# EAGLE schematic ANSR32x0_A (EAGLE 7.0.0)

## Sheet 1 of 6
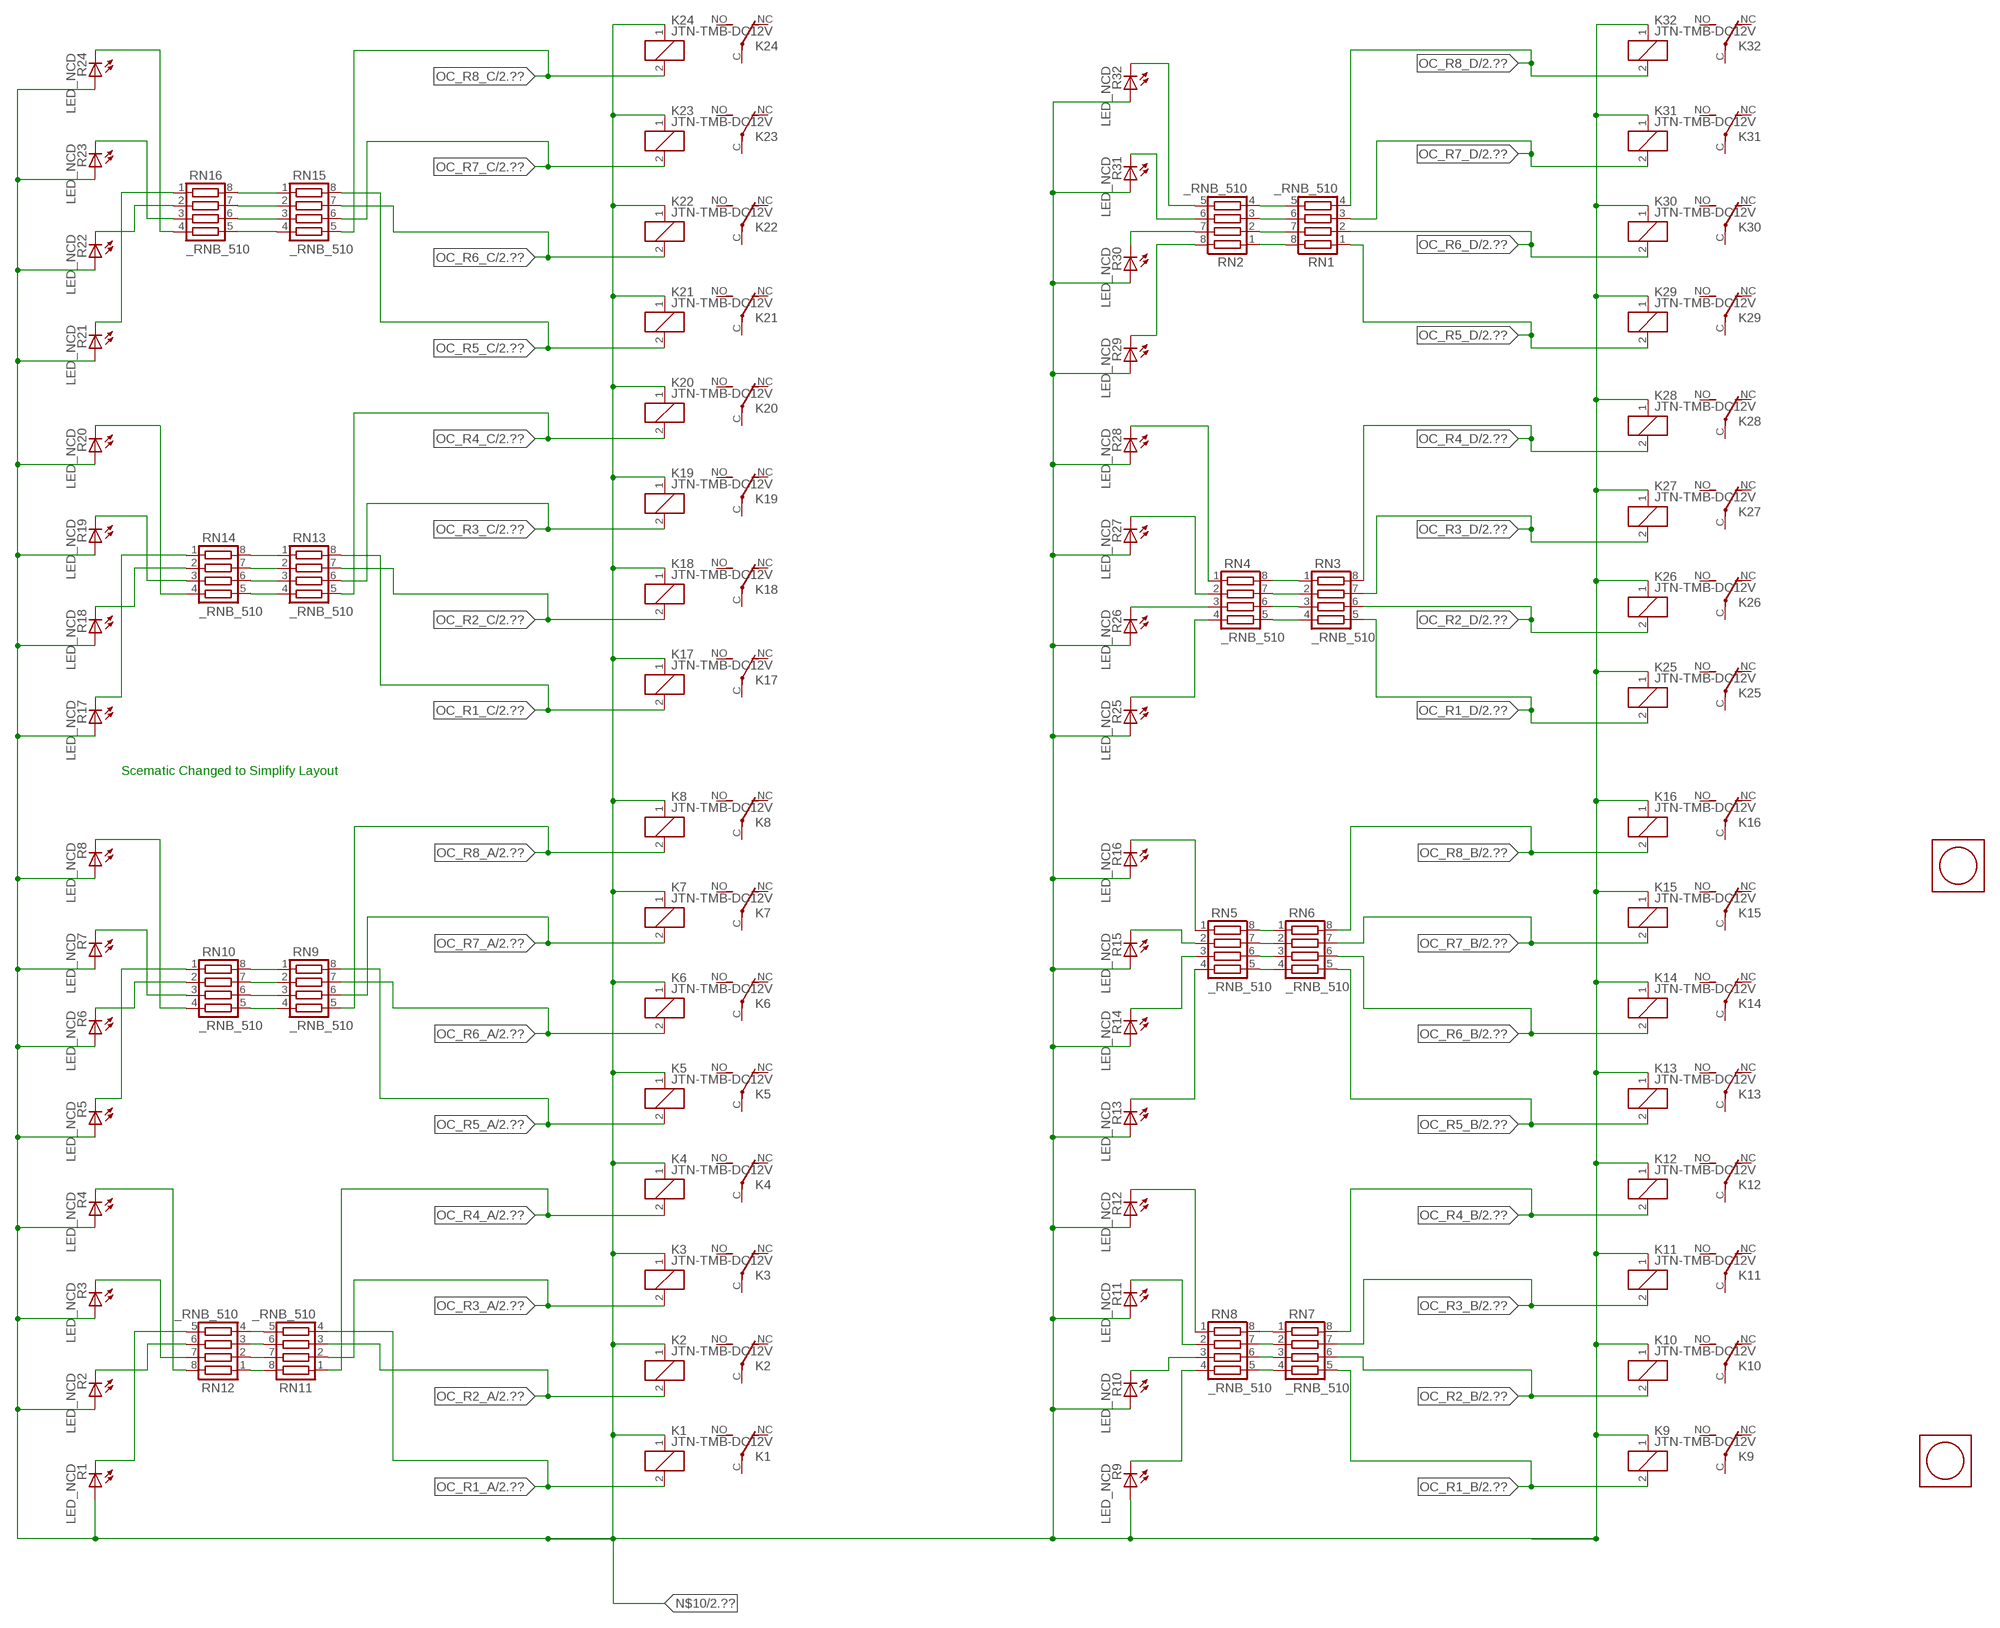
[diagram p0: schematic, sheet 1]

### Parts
K1  JTN-TMB-DC12V  [JT-TMB]
K2  JTN-TMB-DC12V  [JT-TMB]
K3  JTN-TMB-DC12V  [JT-TMB]
K4  JTN-TMB-DC12V  [JT-TMB]
K5  JTN-TMB-DC12V  [JT-TMB]
K6  JTN-TMB-DC12V  [JT-TMB]
K7  JTN-TMB-DC12V  [JT-TMB]
K8  JTN-TMB-DC12V  [JT-TMB]
K9  JTN-TMB-DC12V  [JT-TMB]
K10  JTN-TMB-DC12V  [JT-TMB]
K11  JTN-TMB-DC12V  [JT-TMB]
K12  JTN-TMB-DC12V  [JT-TMB]
K13  JTN-TMB-DC12V  [JT-TMB]
K14  JTN-TMB-DC12V  [JT-TMB]
K15  JTN-TMB-DC12V  [JT-TMB]
K16  JTN-TMB-DC12V  [JT-TMB]
K17  JTN-TMB-DC12V  [JT-TMB]
K18  JTN-TMB-DC12V  [JT-TMB]
K19  JTN-TMB-DC12V  [JT-TMB]
K20  JTN-TMB-DC12V  [JT-TMB]
K21  JTN-TMB-DC12V  [JT-TMB]
K22  JTN-TMB-DC12V  [JT-TMB]
K23  JTN-TMB-DC12V  [JT-TMB]
K24  JTN-TMB-DC12V  [JT-TMB]
K25  JTN-TMB-DC12V  [JT-TMB]
K26  JTN-TMB-DC12V  [JT-TMB]
K27  JTN-TMB-DC12V  [JT-TMB]
K28  JTN-TMB-DC12V  [JT-TMB]
K29  JTN-TMB-DC12V  [JT-TMB]
K30  JTN-TMB-DC12V  [JT-TMB]
K31  JTN-TMB-DC12V  [JT-TMB]
K32  JTN-TMB-DC12V  [JT-TMB]
R1  LED_NCD  [CHIPLED_0603]
R2  LED_NCD  [CHIPLED_0603]
R3  LED_NCD  [CHIPLED_0603]
R4  LED_NCD  [CHIPLED_0603]
R5  LED_NCD  [CHIPLED_0603]
R6  LED_NCD  [CHIPLED_0603]
R7  LED_NCD  [CHIPLED_0603]
R8  LED_NCD  [CHIPLED_0603]
R9  LED_NCD  [CHIPLED_0603]
R10  LED_NCD  [CHIPLED_0603]
R11  LED_NCD  [CHIPLED_0603]
R12  LED_NCD  [CHIPLED_0603]
R13  LED_NCD  [CHIPLED_0603]
R14  LED_NCD  [CHIPLED_0603]
R15  LED_NCD  [CHIPLED_0603]
R16  LED_NCD  [CHIPLED_0603]
R17  LED_NCD  [CHIPLED_0603]
R18  LED_NCD  [CHIPLED_0603]
R19  LED_NCD  [CHIPLED_0603]
R20  LED_NCD  [CHIPLED_0603]
R21  LED_NCD  [CHIPLED_0603]
R22  LED_NCD  [CHIPLED_0603]
R23  LED_NCD  [CHIPLED_0603]
R24  LED_NCD  [CHIPLED_0603]
R25  LED_NCD  [CHIPLED_0603]
R26  LED_NCD  [CHIPLED_0603]
R27  LED_NCD  [CHIPLED_0603]
R28  LED_NCD  [CHIPLED_0603]
R29  LED_NCD  [CHIPLED_0603]
R30  LED_NCD  [CHIPLED_0603]
R31  LED_NCD  [CHIPLED_0603]
R32  LED_NCD  [CHIPLED_0603]
RN1  _RNB_510  [RNB]
RN2  _RNB_510  [RNB]
RN3  _RNB_510  [RNB]
RN4  _RNB_510  [RNB]
RN5  _RNB_510  [RNB]
RN6  _RNB_510  [RNB]
RN7  _RNB_510  [RNB]
RN8  _RNB_510  [RNB]
RN9  _RNB_510  [RNB]
RN10  _RNB_510  [RNB]
RN11  _RNB_510  [RNB]
RN12  _RNB_510  [RNB]
RN13  _RNB_510  [RNB]
RN14  _RNB_510  [RNB]
RN15  _RNB_510  [RNB]
RN16  _RNB_510  [RNB]
U$1  PCB_MOUNTING_HOLE  [PCB_MOUNTING_HOLE]
U$3  PCB_MOUNTING_HOLE  [PCB_MOUNTING_HOLE]

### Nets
N$10: K1.1(C1) K2.1(C1) K3.1(C1) K4.1(C1) K5.1(C1) K6.1(C1) K7.1(C1) K8.1(C1) K9.1(C1) K10.1(C1) K11.1(C1) K12.1(C1) K13.1(C1) K14.1(C1) K15.1(C1) K16.1(C1) K17.1(C1) K18.1(C1) K19.1(C1) K20.1(C1) K21.1(C1) K22.1(C1) K23.1(C1) K24.1(C1) K25.1(C1) K26.1(C1) K27.1(C1) K28.1(C1) K29.1(C1) K30.1(C1) K31.1(C1) K32.1(C1) R1.A R2.A R3.A R4.A R5.A R6.A R7.A R8.A R9.A R10.A R11.A R12.A R13.A R14.A R15.A R16.A R17.A R18.A R19.A R20.A R21.A R22.A R23.A R24.A R25.A R26.A R27.A R28.A R29.A R30.A R31.A R32.A ; also sheet 2
N$440: R30.C RN2.7
N$441: R16.C RN5.1
N$442: RN7.2 RN8.7
N$443: RN7.3 RN8.6
N$444: RN7.4 RN8.5
N$445: R15.C RN5.2
N$446: R26.C RN4.3
N$447: R13.C RN5.4
N$448: RN5.5 RN6.4
N$449: RN7.1 RN8.8
N$450: R12.C RN8.1
N$451: RN5.6 RN6.3
N$452: R11.C RN8.2
N$453: RN5.7 RN6.2
N$454: RN5.8 RN6.1
N$455: RN3.4 RN4.5
N$456: R32.C RN2.5
N$458: R14.C RN5.3
N$459: R10.C RN8.3
N$460: R29.C RN2.8
N$461: R28.C RN4.1
N$462: R27.C RN4.2
N$463: RN11.5 RN12.4
N$464: R25.C RN4.4
N$465: RN1.8 RN2.1
N$466: RN1.7 RN2.2
N$467: RN1.6 RN2.3
N$468: RN1.5 RN2.4
N$469: R31.C RN2.6
N$470: R9.C RN8.4
N$473: R1.C RN12.5
N$474: RN11.6 RN12.3
N$475: R2.C RN12.6
N$476: R3.C RN12.7
N$477: RN9.4 RN10.5
N$478: RN9.3 RN10.6
N$479: RN9.2 RN10.7
N$480: RN9.1 RN10.8
N$481: RN11.7 RN12.2
N$482: R5.C RN10.1
N$483: R4.C RN12.8
N$484: R7.C RN10.3
N$485: R8.C RN10.4
N$486: R6.C RN10.2
N$487: R19.C RN14.3
N$488: R18.C RN14.2
N$489: R17.C RN14.1
N$490: R24.C RN16.4
N$491: RN15.3 RN16.6
N$492: RN15.2 RN16.7
N$493: RN15.1 RN16.8
N$494: R20.C RN14.4
N$495: R23.C RN16.3
N$496: R22.C RN16.2
N$497: R21.C RN16.1
N$500: RN11.8 RN12.1
N$501: RN13.4 RN14.5
N$502: RN13.3 RN14.6
N$503: RN13.2 RN14.7
N$504: RN13.1 RN14.8
N$505: RN3.3 RN4.6
N$506: RN3.2 RN4.7
N$507: RN3.1 RN4.8
N$514: RN15.4 RN16.5
OC_R1_A: K1.2(C2) RN11.4 ; also sheet 2
OC_R1_B: K9.2(C2) RN7.5 ; also sheet 2
OC_R1_C: K17.2(C2) RN13.8 ; also sheet 2
OC_R1_D: K25.2(C2) RN3.5 ; also sheet 2
OC_R2_A: K2.2(C2) RN11.3 ; also sheet 2
OC_R2_B: K10.2(C2) RN7.6 ; also sheet 2
OC_R2_C: K18.2(C2) RN13.7 ; also sheet 2
OC_R2_D: K26.2(C2) RN3.6 ; also sheet 2
OC_R3_A: K3.2(C2) RN11.2 ; also sheet 2
OC_R3_B: K11.2(C2) RN7.7 ; also sheet 2
OC_R3_C: K19.2(C2) RN13.6 ; also sheet 2
OC_R3_D: K27.2(C2) RN3.7 ; also sheet 2
OC_R4_A: K4.2(C2) RN11.1 ; also sheet 2
OC_R4_B: K12.2(C2) RN7.8 ; also sheet 2
OC_R4_C: K20.2(C2) RN13.5 ; also sheet 2
OC_R4_D: K28.2(C2) RN3.8 ; also sheet 2
OC_R5_A: K5.2(C2) RN9.8 ; also sheet 2
OC_R5_B: K13.2(C2) RN6.5 ; also sheet 2
OC_R5_C: K21.2(C2) RN15.8 ; also sheet 2
OC_R5_D: K29.2(C2) RN1.1 ; also sheet 2
OC_R6_A: K6.2(C2) RN9.7 ; also sheet 2
OC_R6_B: K14.2(C2) RN6.6 ; also sheet 2
OC_R6_C: K22.2(C2) RN15.7 ; also sheet 2
OC_R6_D: K30.2(C2) RN1.2 ; also sheet 2
OC_R7_A: K7.2(C2) RN9.6 ; also sheet 2
OC_R7_B: K15.2(C2) RN6.7 ; also sheet 2
OC_R7_C: K23.2(C2) RN15.6 ; also sheet 2
OC_R7_D: K31.2(C2) RN1.3 ; also sheet 2
OC_R8_A: K8.2(C2) RN9.5 ; also sheet 2
OC_R8_B: K16.2(C2) RN6.8 ; also sheet 2
OC_R8_C: K24.2(C2) RN15.5 ; also sheet 2
OC_R8_D: K32.2(C2) RN1.4 ; also sheet 2
Unconnected: K1.C(COM) K1.NC K1.NO K2.C(COM) K2.NC K2.NO K3.C(COM) K3.NC K3.NO K4.C(COM) K4.NC K4.NO K5.C(COM) K5.NC K5.NO K6.C(COM) K6.NC K6.NO K7.C(COM) K7.NC K7.NO K8.C(COM) K8.NC K8.NO K9.C(COM) K9.NC K9.NO K10.C(COM) K10.NC K10.NO K11.C(COM) K11.NC K11.NO K12.C(COM) K12.NC K12.NO K13.C(COM) K13.NC K13.NO K14.C(COM) K14.NC K14.NO K15.C(COM) K15.NC K15.NO K16.C(COM) K16.NC K16.NO K17.C(COM) K17.NC K17.NO K18.C(COM) K18.NC K18.NO K19.C(COM) K19.NC K19.NO K20.C(COM) K20.NC K20.NO K21.C(COM) K21.NC K21.NO K22.C(COM) K22.NC K22.NO K23.C(COM) K23.NC K23.NO K24.C(COM) K24.NC K24.NO K25.C(COM) K25.NC K25.NO K26.C(COM) K26.NC K26.NO K27.C(COM) K27.NC K27.NO K28.C(COM) K28.NC K28.NO K29.C(COM) K29.NC K29.NO K30.C(COM) K30.NC K30.NO K31.C(COM) K31.NC K31.NO K32.C(COM) K32.NC K32.NO

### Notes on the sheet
- Scematic Changed to Simplify Layout

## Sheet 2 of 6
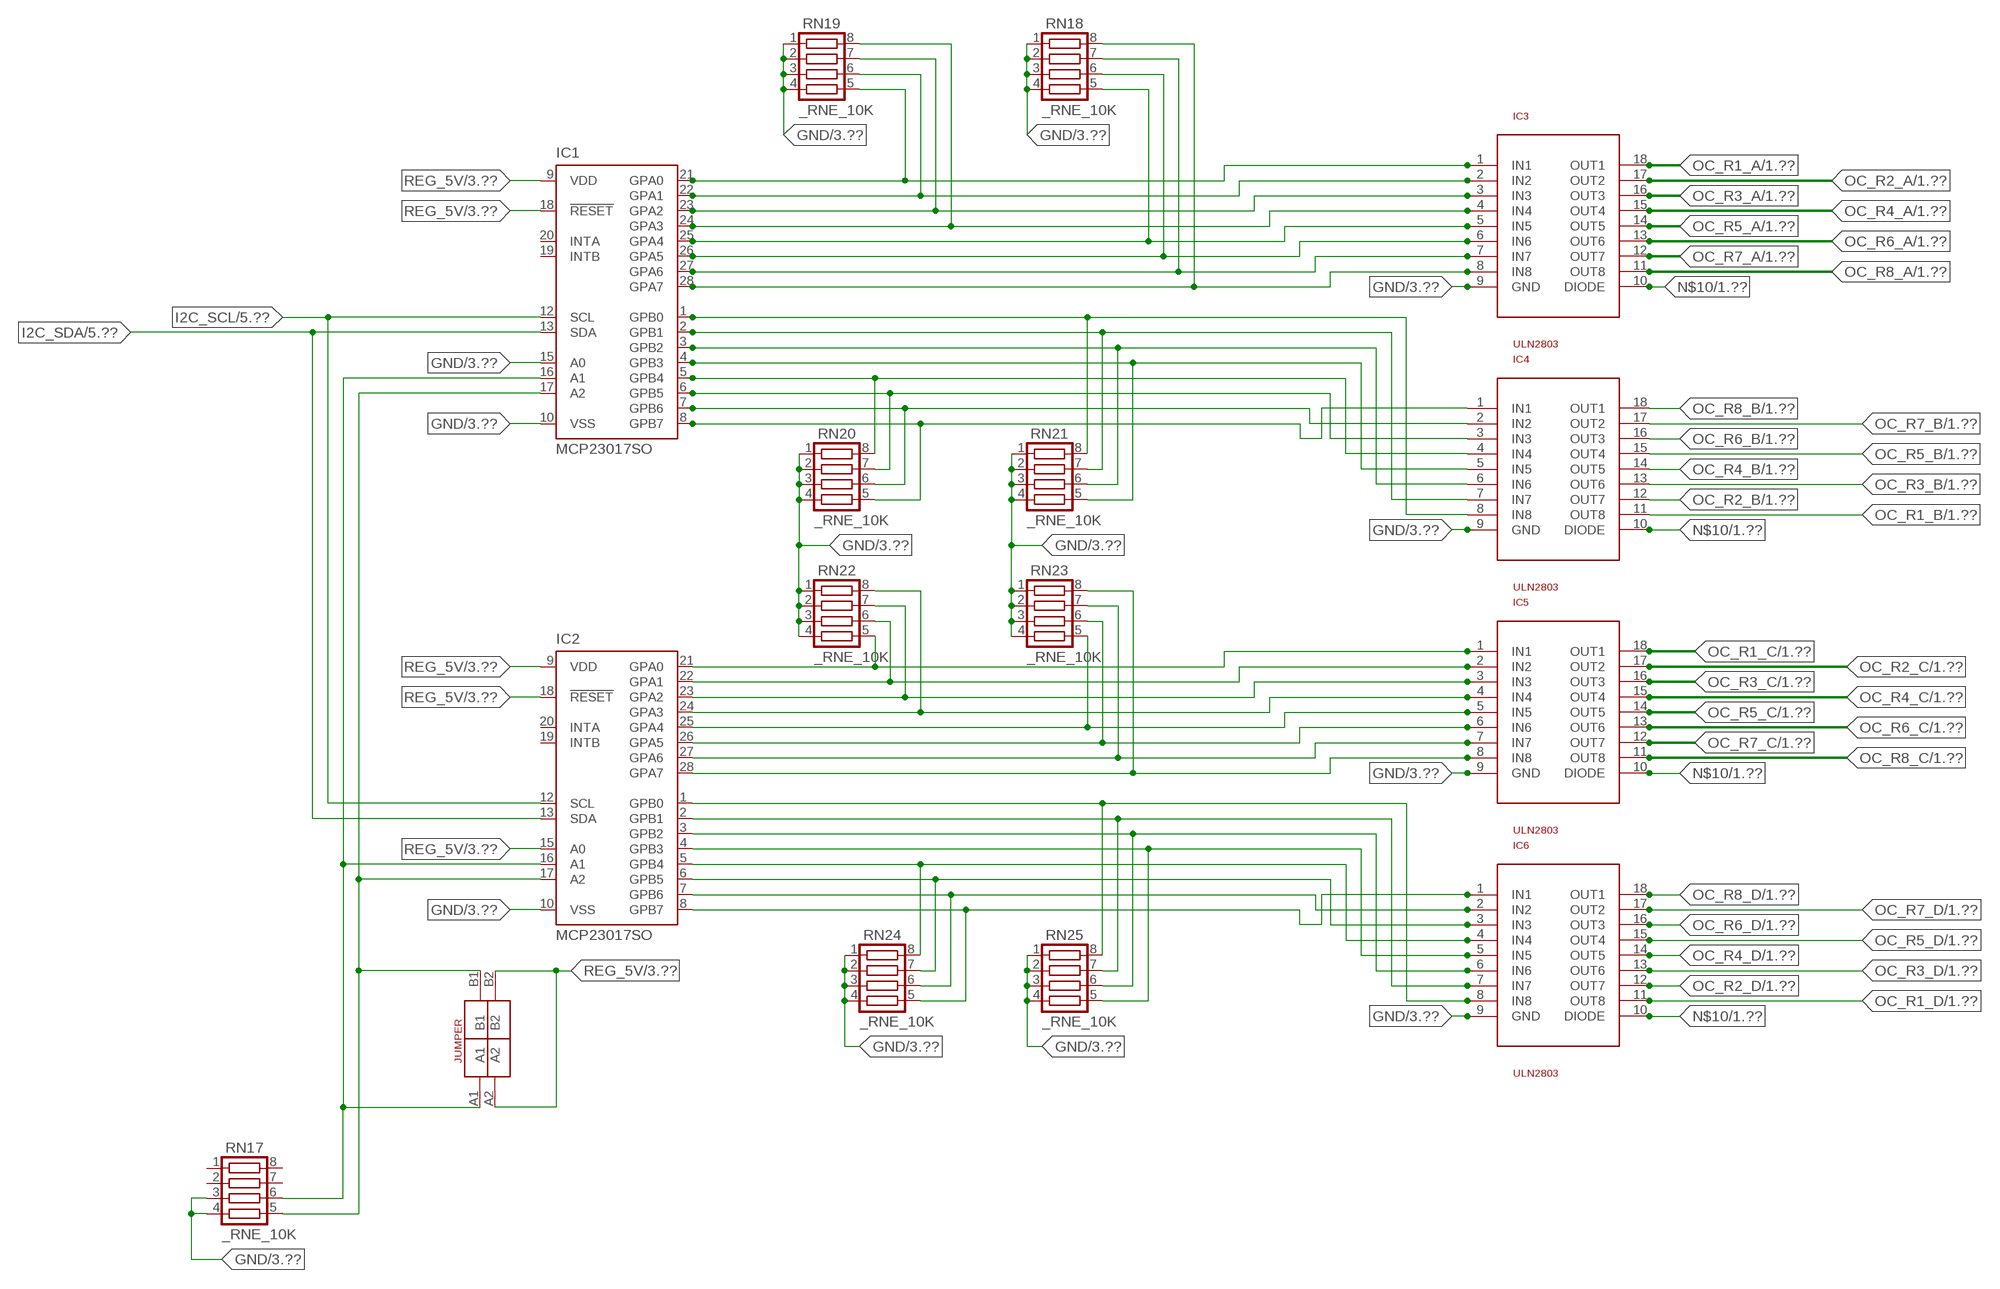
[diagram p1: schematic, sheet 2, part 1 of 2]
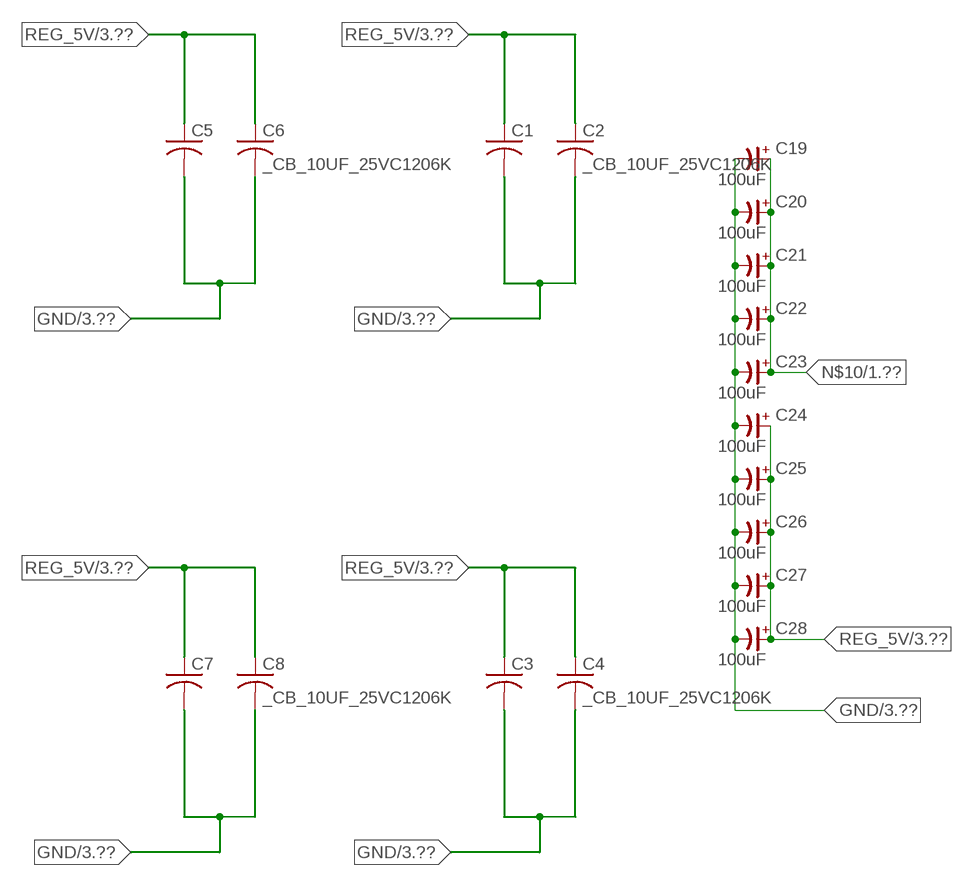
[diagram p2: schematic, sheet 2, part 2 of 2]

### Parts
C1  _CA_.10UF_50VC1206K  [_CA_.1UF_50V]
C2  _CB_10UF_25VC1206K  [_CB_10UF_25V]
C3  _CA_.10UF_50VC1206K  [_CA_.1UF_50V]
C4  _CB_10UF_25VC1206K  [_CB_10UF_25V]
C5  _CA_.10UF_50VC1206K  [_CA_.1UF_50V]
C6  _CB_10UF_25VC1206K  [_CB_10UF_25V]
C7  _CA_.10UF_50VC1206K  [_CA_.1UF_50V]
C8  _CB_10UF_25VC1206K  [_CB_10UF_25V]
C19  100uF  CP-E-025X060  [E-025X060]
C20  100uF  CP-E-025X060  [E-025X060]
C21  100uF  CP-E-025X060  [E-025X060]
C22  100uF  CP-E-025X060  [E-025X060]
C23  100uF  CP-E-025X060  [E-025X060]
C24  100uF  CP-E-025X060  [E-025X060]
C25  100uF  CP-E-025X060  [E-025X060]
C26  100uF  CP-E-025X060  [E-025X060]
C27  100uF  CP-E-025X060  [E-025X060]
C28  100uF  CP-E-025X060  [E-025X060]
IC1  MCP23017SO  [SO28W]
IC2  MCP23017SO  [SO28W]
IC3  ULN2803  [SO18L]
IC4  ULN2803  [SO18L]
IC5  ULN2803  [SO18L]
IC6  ULN2803  [SO18L]
RN17  _RNE_10K  [RNE]
RN18  _RNE_10K  [RNE]
RN19  _RNE_10K  [RNE]
RN20  _RNE_10K  [RNE]
RN21  _RNE_10K  [RNE]
RN22  _RNE_10K  [RNE]
RN23  _RNE_10K  [RNE]
RN24  _RNE_10K  [RNE]
RN25  _RNE_10K  [RNE]
U$13  JUMPER_2X2  [JUMPER_2X2]

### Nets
GND: C1.2 C2.2 C3.2 C4.2 C5.2 C6.2 C7.2 C8.2 C19.- C20.- C21.- C22.- C23.- C24.- C25.- C26.- C27.- C28.- IC1.10(VSS) IC1.15(A0) IC2.10(VSS) IC3.9(GND) IC4.9(GND) IC5.9(GND) IC6.9(GND) RN17.3 RN17.4 RN18.1 RN18.2 RN18.3 RN18.4 RN19.1 RN19.2 RN19.3 RN19.4 RN20.1 RN20.2 RN20.3 RN20.4 RN21.1 RN21.2 RN21.3 RN21.4 RN22.1 RN22.2 RN22.3 RN22.4 RN23.1 RN23.2 RN23.3 RN23.4 RN24.1 RN24.2 RN24.3 RN24.4 RN25.1 RN25.2 RN25.3 RN25.4 ; also sheet 3,4,5,6
I2C_SCL: IC1.12(SCL) IC2.12(SCL) ; also sheet 5,6
I2C_SDA: IC1.13(SDA) IC2.13(SDA) ; also sheet 5,6
N$10: C19.+ C20.+ C21.+ C22.+ C23.+ IC3.10(DIODE) IC4.10(DIODE) IC5.10(DIODE) IC6.10(DIODE) ; also sheet 1
N$405: IC1.21(GPA0) IC3.1(IN1) RN19.5
N$406: IC1.25(GPA4) IC3.5(IN5) RN18.5
N$407: IC1.26(GPA5) IC3.6(IN6) RN18.6
N$408: IC1.16(A1) IC2.16(A1) RN17.6 U$13.A1
N$409: IC1.22(GPA1) IC3.2(IN2) RN19.6
N$410: IC1.23(GPA2) IC3.3(IN3) RN19.7
N$411: IC1.24(GPA3) IC3.4(IN4) RN19.8
N$416: IC1.1(GPB0) IC4.8(IN8) RN21.8
N$417: IC1.2(GPB1) IC4.7(IN7) RN21.7
N$418: IC1.3(GPB2) IC4.6(IN6) RN21.6
N$419: IC1.4(GPB3) IC4.5(IN5) RN21.5
N$420: IC1.5(GPB4) IC4.4(IN4) RN20.8
N$421: IC1.6(GPB5) IC4.3(IN3) RN20.7
N$422: IC1.7(GPB6) IC4.2(IN2) RN20.6
N$423: IC1.8(GPB7) IC4.1(IN1) RN20.5
N$424: IC2.21(GPA0) IC5.1(IN1) RN22.5
N$425: IC2.22(GPA1) IC5.2(IN2) RN22.6
N$426: IC2.23(GPA2) IC5.3(IN3) RN22.7
N$427: IC2.24(GPA3) IC5.4(IN4) RN22.8
N$428: IC2.25(GPA4) IC5.5(IN5) RN23.5
N$429: IC2.26(GPA5) IC5.6(IN6) RN23.6
N$430: IC2.27(GPA6) IC5.7(IN7) RN23.7
N$431: IC2.28(GPA7) IC5.8(IN8) RN23.8
N$432: IC2.1(GPB0) IC6.8(IN8) RN25.8
N$433: IC2.2(GPB1) IC6.7(IN7) RN25.7
N$434: IC2.3(GPB2) IC6.6(IN6) RN25.6
N$435: IC2.4(GPB3) IC6.5(IN5) RN25.5
N$436: IC2.5(GPB4) IC6.4(IN4) RN24.8
N$437: IC2.6(GPB5) IC6.3(IN3) RN24.7
N$438: IC2.7(GPB6) IC6.2(IN2) RN24.6
N$439: IC2.8(GPB7) IC6.1(IN1) RN24.5
N$498: IC1.17(A2) IC2.17(A2) RN17.5 U$13.B1
N$525: IC1.27(GPA6) IC3.7(IN7) RN18.7
N$526: IC1.28(GPA7) IC3.8(IN8) RN18.8
OC_R1_A: IC3.18(OUT1) ; also sheet 1
OC_R1_B: IC4.11(OUT8) ; also sheet 1
OC_R1_C: IC5.18(OUT1) ; also sheet 1
OC_R1_D: IC6.11(OUT8) ; also sheet 1
OC_R2_A: IC3.17(OUT2) ; also sheet 1
OC_R2_B: IC4.12(OUT7) ; also sheet 1
OC_R2_C: IC5.17(OUT2) ; also sheet 1
OC_R2_D: IC6.12(OUT7) ; also sheet 1
OC_R3_A: IC3.16(OUT3) ; also sheet 1
OC_R3_B: IC4.13(OUT6) ; also sheet 1
OC_R3_C: IC5.16(OUT3) ; also sheet 1
OC_R3_D: IC6.13(OUT6) ; also sheet 1
OC_R4_A: IC3.15(OUT4) ; also sheet 1
OC_R4_B: IC4.14(OUT5) ; also sheet 1
OC_R4_C: IC5.15(OUT4) ; also sheet 1
OC_R4_D: IC6.14(OUT5) ; also sheet 1
OC_R5_A: IC3.14(OUT5) ; also sheet 1
OC_R5_B: IC4.15(OUT4) ; also sheet 1
OC_R5_C: IC5.14(OUT5) ; also sheet 1
OC_R5_D: IC6.15(OUT4) ; also sheet 1
OC_R6_A: IC3.13(OUT6) ; also sheet 1
OC_R6_B: IC4.16(OUT3) ; also sheet 1
OC_R6_C: IC5.13(OUT6) ; also sheet 1
OC_R6_D: IC6.16(OUT3) ; also sheet 1
OC_R7_A: IC3.12(OUT7) ; also sheet 1
OC_R7_B: IC4.17(OUT2) ; also sheet 1
OC_R7_C: IC5.12(OUT7) ; also sheet 1
OC_R7_D: IC6.17(OUT2) ; also sheet 1
OC_R8_A: IC3.11(OUT8) ; also sheet 1
OC_R8_B: IC4.18(OUT1) ; also sheet 1
OC_R8_C: IC5.11(OUT8) ; also sheet 1
OC_R8_D: IC6.18(OUT1) ; also sheet 1
REG_5V: C1.1 C2.1 C3.1 C4.1 C5.1 C6.1 C7.1 C8.1 C24.+ C25.+ C26.+ C27.+ C28.+ IC1.9(VDD) IC1.18(!RESET) IC2.9(VDD) IC2.15(A0) IC2.18(!RESET) U$13.A2 U$13.B2 ; also sheet 3,4,5,6
Unconnected: IC1.19(INTB) IC1.20(INTA) IC2.19(INTB) IC2.20(INTA) RN17.1 RN17.2 RN17.7 RN17.8

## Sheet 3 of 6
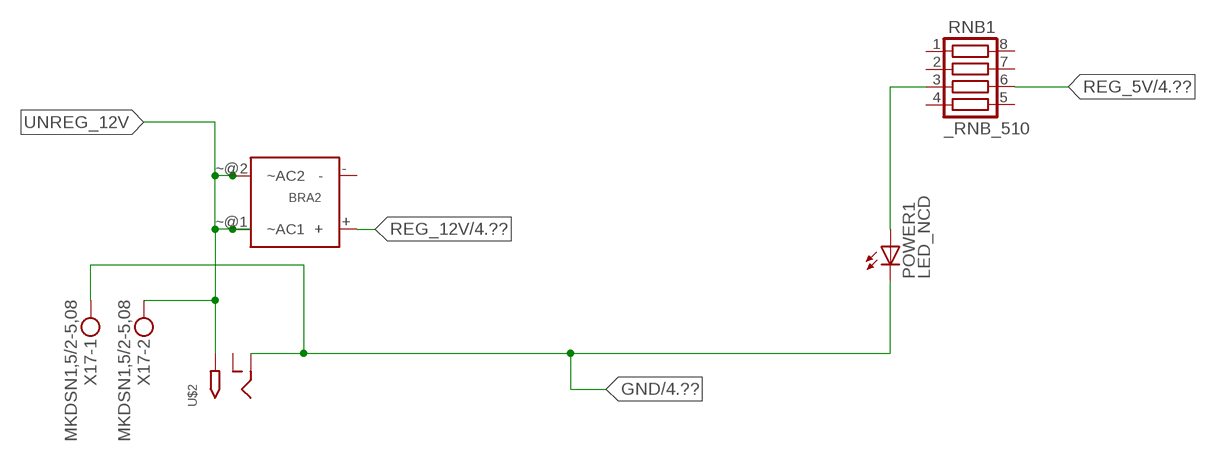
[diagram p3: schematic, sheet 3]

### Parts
BRA2  MB2S_  [MB2S]
POWER1  LED_NCD  [CHIPLED_0603]
RNB1  _RNB_510  [RNB]
U$2  2.1MMJACK  [PJ-102A]
X17  MKDSN1,5/2-5,08  [MKDSN1,5/2-5,08]

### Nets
GND: POWER1.C U$2.RING X17.1 ; also sheet 2,4,5,6
N$99: POWER1.A RNB1.3
REG_5V: RNB1.6 ; also sheet 2,4,5,6
REG_12V: BRA2.+ ; also sheet 4
UNREG_12V: BRA2.~@1(~AC1) BRA2.~@2(~AC2) U$2.TIP X17.2
Unconnected: BRA2.- RNB1.1 RNB1.2 RNB1.4 RNB1.5 RNB1.7 RNB1.8 U$2.RING_SW

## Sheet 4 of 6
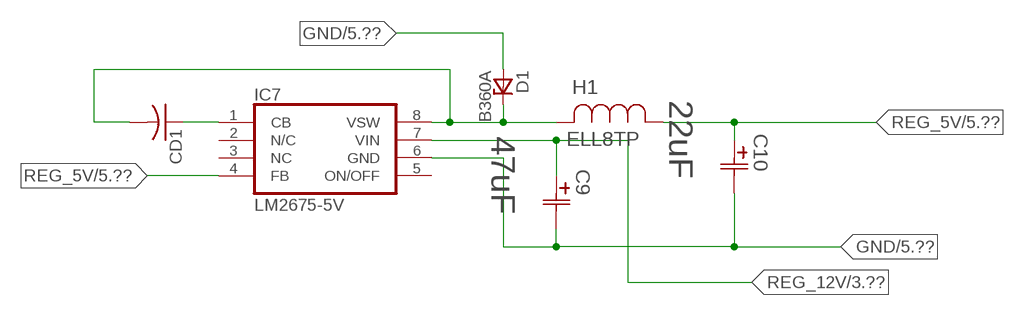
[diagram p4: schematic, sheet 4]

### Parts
C9  47uF  490-5463-6-NDCAP  [C2917(7343)-Y]
C10  22uF  490-5463-6-NDCAP  [C2917(7343)-Y]
CD1  _CD_10NF_50VC1206K  [_CD_10NF_50V]
D1  B360A  [DO214AC_ZENER]
H1  ELL8TP  [IND_ELL8TP]
IC7  LM2675-5V  LM2675  [SO-8]

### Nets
GND: C9.2(C2) C10.2(C2) D1.A IC7.6(GND) ; also sheet 2,3,5,6
N$100: CD1.2 D1.C H1.2 IC7.8(VSW)
N$101: CD1.1 IC7.1(CB)
REG_5V: C10.1(C1) H1.1 IC7.4(FB) ; also sheet 2,3,5,6
REG_12V: C9.1(C1) IC7.7(VIN) ; also sheet 3
Unconnected: IC7.2(N/C) IC7.5(ON/OFF)

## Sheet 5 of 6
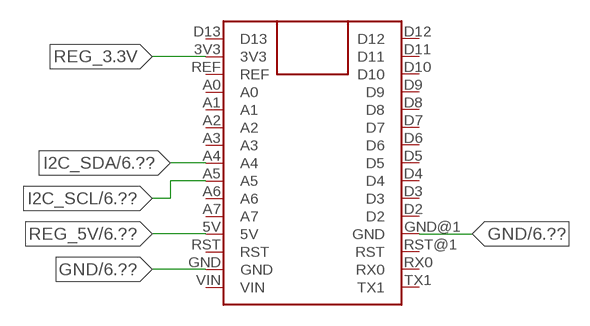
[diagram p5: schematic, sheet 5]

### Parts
FOR_NANO  ARDUINO_NANO  [ARDUINO_NANO]

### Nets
GND: FOR_NANO.GND FOR_NANO.GND@1(GND) ; also sheet 2,3,4,6
I2C_SCL: FOR_NANO.A5 ; also sheet 2,6
I2C_SDA: FOR_NANO.A4 ; also sheet 2,6
REG_3.3V: FOR_NANO.3V3
REG_5V: FOR_NANO.5V ; also sheet 2,3,4,6
Unconnected: FOR_NANO.A0 FOR_NANO.A1 FOR_NANO.A2 FOR_NANO.A3 FOR_NANO.A6 FOR_NANO.A7 FOR_NANO.D2 FOR_NANO.D3 FOR_NANO.D4 FOR_NANO.D5 FOR_NANO.D6 FOR_NANO.D7 FOR_NANO.D8 FOR_NANO.D9 FOR_NANO.D10 FOR_NANO.D11 FOR_NANO.D12 FOR_NANO.D13 FOR_NANO.REF FOR_NANO.RST FOR_NANO.RST@1(RST) FOR_NANO.RX0 FOR_NANO.TX1 FOR_NANO.VIN

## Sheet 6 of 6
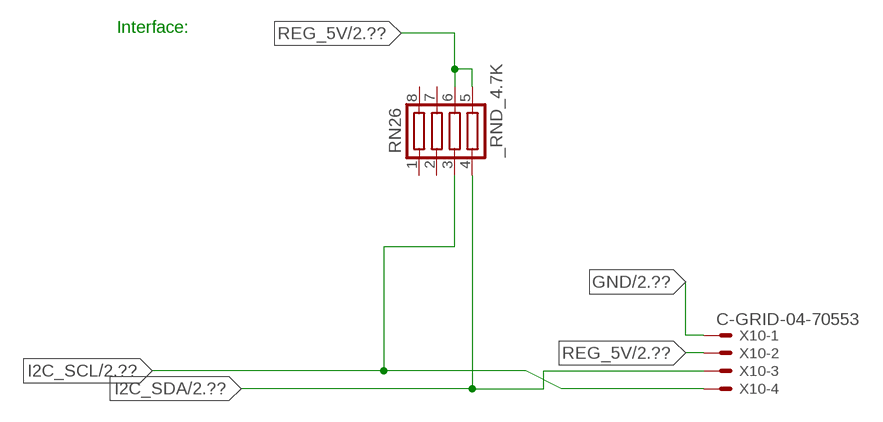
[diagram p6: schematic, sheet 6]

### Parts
RN26  _RND_4.7K  [RND]
X10  C-GRID-04-70553  [70553-04]

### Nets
GND: X10.1 ; also sheet 2,3,4,5
I2C_SCL: RN26.3 X10.4 ; also sheet 2,5
I2C_SDA: RN26.4 X10.3 ; also sheet 2,5
REG_5V: RN26.5 RN26.6 X10.2 ; also sheet 2,3,4,5
Unconnected: RN26.1 RN26.2 RN26.7 RN26.8

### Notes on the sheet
- Interface:

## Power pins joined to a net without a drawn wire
NC: IC7.3(NC)

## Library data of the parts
BRA2 = NCD_ULTIMATE_LIBRARY:MB2S: Bridge Rectifier BRA MB2S 200V 500ma Digikey MB2S-TPMSTR-ND/MB2S-TP
C1 C3 C5 C7 = NCD_ULTIMATE_LIBRARY:_CA_.10UF_50V: Capacitor .1uF SMT
C2 C4 C6 C8 = NCD_ULTIMATE_LIBRARY:_CB_10UF_25V: Capacitor 10uF SMT
C9 C10 = NCD_ULTIMATE_bhaskar:490-5463-6-ND: NCD CAP
C19-C28 = NCD_ULTIMATE_LIBRARY:CP-: Capacitors All Kinds POLARIZED CAP
CD1 = NCD_ULTIMATE_LIBRARY:_CD_10NF_50V: Capacitor 10nF SMT
D1 = NCD_ULTIMATE_bhaskar:B360A: NCD DIODE B350A/B360A
FOR_NANO = NCD_ULTIMATE_CONNECTORS:ARDUINO_NANO
H1 = NCD_ULTIMATE_bhaskar:ELL8TP: NCD coil
IC1 IC2 = NCD_ULTIMATE_LIBRARY:MCP23017: Semiconductor Port Expander I/O 16-Bit I2C http://ww1.microchip.com/downloads/en/DeviceDoc/21952a.pdf Source: http://ww1.microchip.com/downloads/en/DeviceDoc/21952a.pdf
IC3-IC6 = NCD_ULTIMATE_LIBRARY:ULN2803: Semiconductor 8 O.C. N-Channel Transistor Driver Digikey ULN2803AFWGCELTR-ND/ULN2803AFWG,C,EL
IC7 = NCD_ULTIMATE_bhaskar:LM2675: LM2675 NCD http://www.ti.com/lit/ds/symlink/lm2675.pdf
K1-K32 = NCD_ULTIMATE_LIBRARY:JT?-*: RELAY COMPACT ECONOMICAL 30 AMP. RELAY NAiS Source: http://www.mew-europe.com/.. en_ds_61212_0000.pdf
POWER1 R1-R32 = NCD_ULTIMATE_bhaskar:LED_NCD
RN1-RN16 RNB1 = NCD_ULTIMATE_LIBRARY:_RNB_510: Resistor Array RNB SMT 510 x 4 Single Resistor Source: http://www.ctscorp.com/components/Datasheets/CTSChipArrayDs.pdf Digikey 742C083511JPTR-ND/ 742C083511JP; OC_FARNELL: unknown; OC_NEWARK: unknown
RN17-RN25 = NCD_ULTIMATE_LIBRARY:_RNE_10K: Resistor Array RNE SMT 10K x 4 Single Resistor Source: http://www.ctscorp.com/components/Datasheets/CTSChipArrayDs.pdf Digikey 742C083103JPTR-ND/742C083103JP; OC_FARNELL: unknown; OC_NEWARK: unknown
RN26 = NCD_ULTIMATE_LIBRARY:_RND_4.7K: Resistor Array RND SMT 4.7K x 4 Single Resistor Source: http://www.ctscorp.com/components/Datasheets/CTSChipArrayDs.pdf Digikey 742C083472JPTR-ND/742C083472JP; OC_FARNELL: unknown; OC_NEWARK: unknown
U$1 U$3 = NCD_ULTIMATE_CONNECTORS:PCB_MOUNTING_HOLE
U$2 = NCD_ULTIMATE_CONNECTORS:2.1MMJACK: 2.1mm x 5.5mm DC jack with internal switch. Digikey part #PJ-102A, 4UCON part #05537 By microbuilder.eu
U$13 = NCD_ULTIMATE_CONNECTORS:JUMPER_2X2
X10 = NCD_ULTIMATE_CONNECTORS:C-GRID-04: CONNECTOR 4-Pos I2C wire to board 2.54 mm (0.100") pitch header Digikey WM1342-ND/0015912045; OC_FARNELL: unknown; OC_NEWARK: unknown
X17 = NCD_ULTIMATE_CONNECTORS:MKDSN1,5/2-5,08: MKDSN 1,5/ 2-5,08 Printklemme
